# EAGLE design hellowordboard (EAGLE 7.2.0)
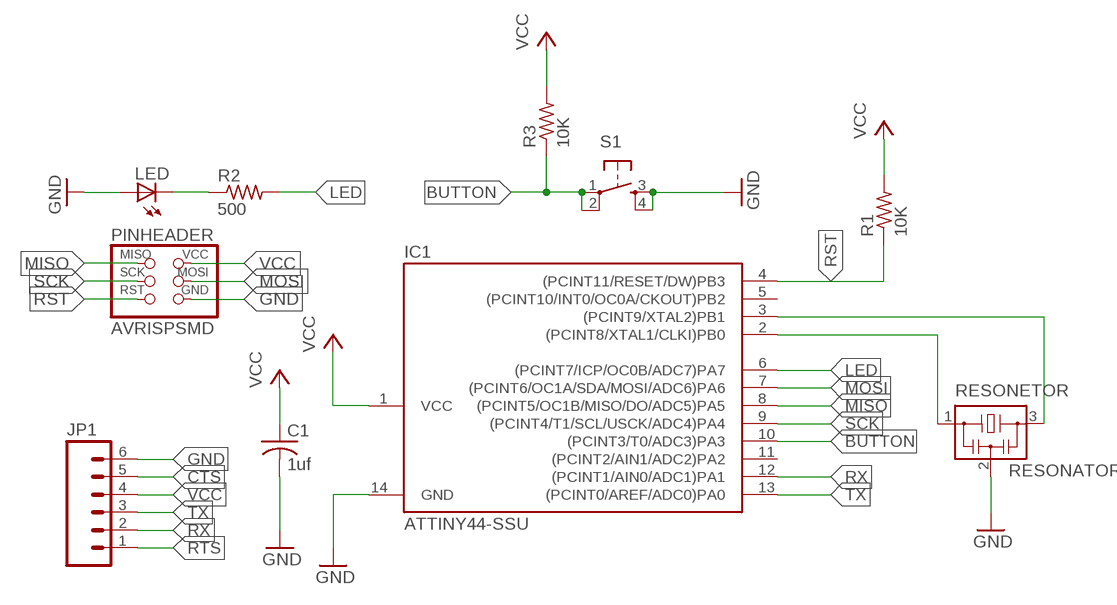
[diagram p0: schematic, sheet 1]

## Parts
C1  1uf  C-USC1206  [C1206]
IC1  ATTINY44-SSU  [SOIC14]
JP1  M06SMD  [1X06-SMD]
LED  LED1206  [1206]
PINHEADER  AVRISPSMD  [2X03SMD]
R1  10K  RESISTOR1206  [1206]
R2  500  RESISTOR1206  [1206]
R3  10K  RESISTOR1206  [1206]
RESONETOR  RESONATOR  [EFOBM]
S1  6MM_SWITCH6MM_SWITCH  [6MM_SWITCH]

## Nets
BUTTON: IC1.10((PCINT3/T0/ADC3)PA3) R3.1 S1.1(P) S1.2(P1)
CTS: JP1.5
GND: C1.2 IC1.14(GND) JP1.6 LED.1(A) PINHEADER.6(GND) RESONETOR.2 S1.3(S) S1.4(S1)
LED: IC1.6((PCINT7/ICP/OC0B/ADC7)PA7) R2.2
MISO: IC1.8((PCINT5/OC1B/MISO/DO/ADC5)PA5) PINHEADER.1(MISO)
MOSI: IC1.7((PCINT6/OC1A/SDA/MOSI/ADC6)PA6) PINHEADER.4(MOSI)
N$2: LED.2(C) R2.1
N$9: IC1.2((PCINT8/XTAL1/CLKI)PB0) RESONETOR.1
N$10: IC1.3((PCINT9/XTAL2)PB1) RESONETOR.3
RST: IC1.4((PCINT11/RESET/DW)PB3) PINHEADER.5(RST) R1.1
RTS: JP1.1
RX: IC1.12((PCINT1/AIN0/ADC1)PA1) JP1.2
SCK: IC1.9((PCINT4/T1/SCL/USCK/ADC4)PA4) PINHEADER.3(SCK)
TX: IC1.13((PCINT0/AREF/ADC0)PA0) JP1.3
VCC: C1.1 IC1.1(VCC) JP1.4 PINHEADER.2(VCC) R1.2 R3.2
Unconnected: IC1.5((PCINT10/INT0/OC0A/CKOUT)PB2) IC1.11((PCINT2/AIN1/ADC2)PA2)

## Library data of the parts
C1 = 01_adafruit:C-US: CAPACITOR, American symbol
IC1 = 01_FAB_Hello:ATTINY44
JP1 = 01_SparkFun:M06: Header 6 Standard 6-pin 0.1" header. Use with straight break away headers (SKU : PRT-00116), right angle break away headers (PRT-00553), swiss pins (PRT-00743), machine pins (PRT-00117), and female headers (PRT-00115). Molex polarized connector foot print use with SKU : PRT-08094 with associated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
LED = 01_FAB_Hello:LED
PINHEADER = 01_FAB_Hello:AVRISP
R1-R3 = 01_FAB_Hello:RESISTOR
RESONETOR = 01_fab:RESONATOR
S1 = 01_FAB_Hello:6MM_SWITCH: OMRON SWITCH

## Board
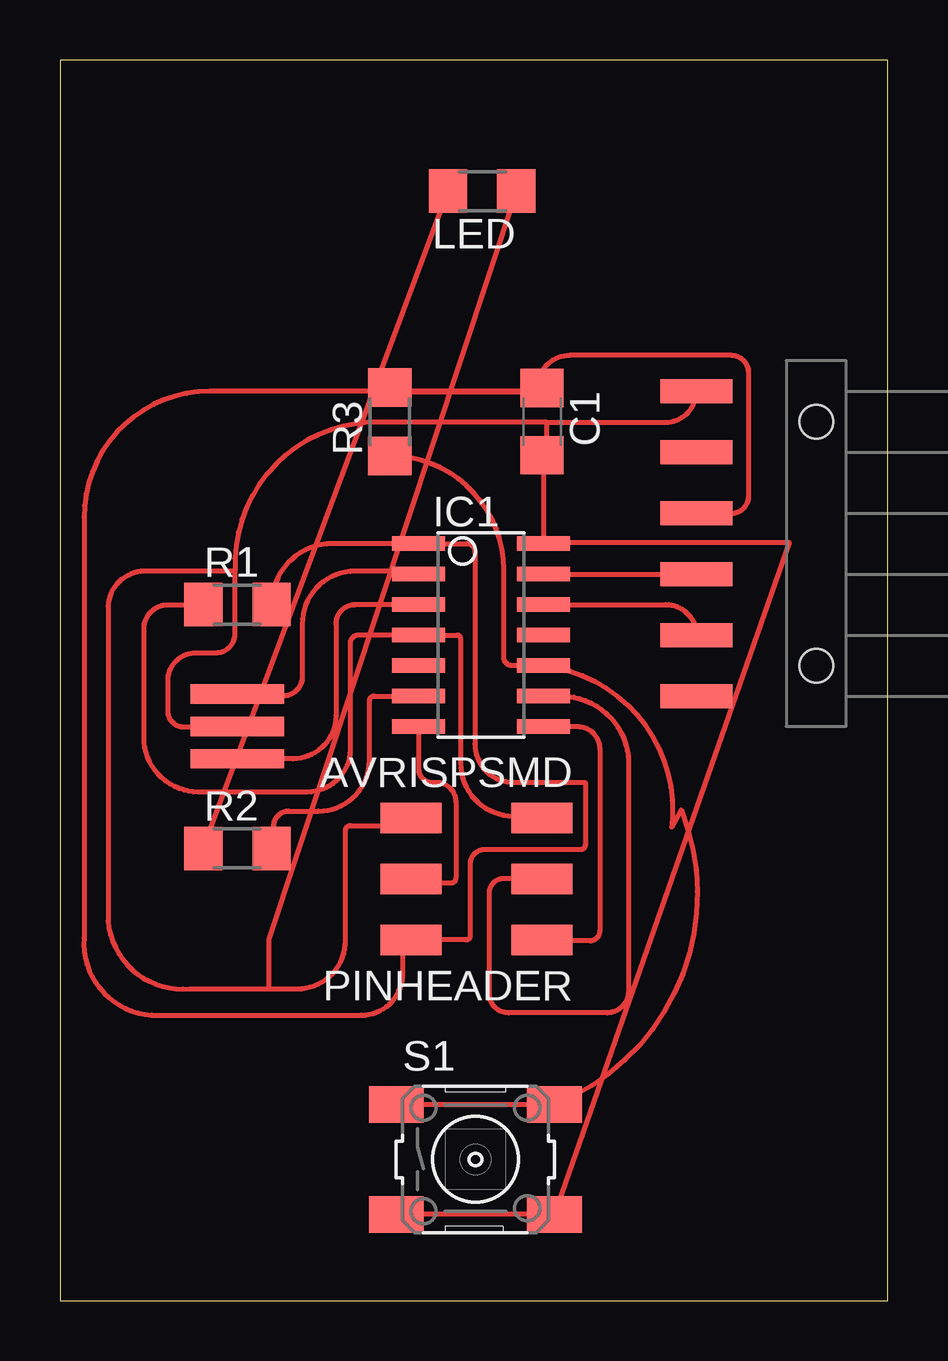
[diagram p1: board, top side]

Size 34.5 x 51.7 mm. Coordinates in mm from the lower left corner, seen from the top.
Outline: 0,0 34.5,0 34.5,51.7 0,51.7 0,0
Copper layers (1*16): Top 0.035mm / dielectric 1.5mm / Bottom 0.035mm
Design rules "default": minimum track width 10mil, minimum drill 24mil, track to track 8mil, track to pad 8mil, pad to pad 8mil, via to via 8mil, smd to smd 8mil, copper to edge 40mil, drill to drill 8mil, minimum pad ring 10mil, minimum via ring 8mil, stop-mask expansion 4mil, vias tented up to drill 0mil, thermal gap 10mil

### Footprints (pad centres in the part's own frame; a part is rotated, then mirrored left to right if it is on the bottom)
C1206 = smd 1.6 x 1.8: 1 -1.4,0; 2 1.4,0
SOIC14 = smd 0.61 x 2.21: 1 -3.81,-2.603; 2 -2.54,-2.603; 3 -1.27,-2.603; 4 0,-2.603; 5 1.27,-2.603; 6 2.54,-2.603; 7 3.81,-2.603; 8 3.81,2.603; 9 2.54,2.603; 10 1.27,2.603; 11 0,2.603; 12 -1.27,2.603; 13 -2.54,2.603; 14 -3.81,2.603
1X06-SMD = smd 1 x 3: 1 -6.35,5; 2 -3.81,5; 3 -1.27,5; 4 1.27,5; 5 3.81,5; 6 6.35,5 | hole 1.4: -5.08,0; 5.08,0
1206 = smd 1.6 x 1.803: 1 -1.422,0; 2 1.422,0
2X03SMD = smd 2.54 x 1.27: 1 -2.54,2.54; 2 2.92,2.54; 3 -2.54,0; 4 2.92,0; 5 -2.54,-2.54; 6 2.92,-2.54
EFOBM = smd 0.8 x 3.9: 1 -1.35,0; 2 0,0; 3 1.35,0
6MM_SWITCH = smd 2.286 x 1.524: 1 -3.302,2.286; 2 3.302,2.286; 3 -3.302,-2.286; 4 3.302,-2.286

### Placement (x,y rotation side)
C1  20.1,36.63 270 top
IC1  17.56,27.74 270 top
JP1  31.53,31.55 90 top
LED  17.6,46.24 180 top
PINHEADER  17.56,17.58 180 top
R1  7.4,29.01 0 top
R2  7.4,18.85 0 top
R3  13.75,36.63 90 top
RESONETOR  7.4,23.93 270 top
S1  17.32,5.89 0 top

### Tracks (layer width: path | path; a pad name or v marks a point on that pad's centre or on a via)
BUTTON
  Top 0.2: S1.1 S1.2 arc90 25.9,20.46 25.5,19.73 arc90 IC1.10 18.83,26.47 arc-90 18.5,26.8 18.5,30.46 arc90 R3.1
  Top 0.254: 13.8,34.9 R3.1
GND
  Top 0.2: 7.3,30.4 arc-90 12.9,36.6 20.3,36.6 | 7.3,30.4 3.65,30.4 arc90 2,28.95 2,15.82 arc90 5.42,13 8.7,13 | S1.3 S1.4 30.41,31.6 20.21,31.6 IC1.14 20.16,35.17 C1.2 | 20.3,35.4 20.3,36.6 | 7.3,23.9 5.17,23.9 arc-90 4.5,24.57 4.5,25.83 arc-90 5.67,27 6.5,27 arc90 7.3,27.8 7.3,30.4 | 20.3,36.6 25.23,36.6 arc90 JP1.6 | 8.7,13 9.9,13 arc90 11.9,15 11.9,19.6 arc-90 12.1,19.8 14.32,19.8 arc90 PINHEADER.6 | LED.1 8.7,15.04 8.7,13
  Top 0.254: 13.8,19.9 14.3,19.9 PINHEADER.6 | 20.3,34.9 C1.2 20.3,35.4 | 7.3,23.9 RESONETOR.2
  Top 0.3: 13.64,19.9 14.64,19.9 PINHEADER.6
LED
  Top 0.2: R2.2 8.9,18.85 8.9,19.77 arc-90 9.53,20.4 10.77,20.4 arc90 12.9,22.53 12.9,25 arc-90 13.1,25.2 IC1.6
MISO
  Top 0.2: IC1.8 21.57,23.93 arc-90 22.5,23 22.5,15.4 arc-90 22.1,15 20.14,15 arc-90 PINHEADER.1
MOSI
  Top 0.2: IC1.7 14.96,22.14 arc90 15.5,21.6 15.7,21.6 arc-90 16.5,20.8 16.5,17.6 arc-90 16.3,17.4 14.82,17.4 arc-90 PINHEADER.4
N$2
  Top 0.2: R2.1 LED.2
N$9
  Top 0.2: 14.8,30.4 12.3,30.4 arc90 10.1,28.2 10.1,26 arc-90 9.3,25.2 7.48,25.2 arc-90 RESONETOR.1
  Top 0.254: 14.8,30.4 IC1.2
N$10
  Top 0.2: IC1.3 arc-90 14.95,29 12.3,29 arc90 11.5,28.2 11.5,24.38 arc-90 9.7,22.58 RESONETOR.3
RST
  Top 0.2: PINHEADER.5 arc90 20.02,20.2 18.9,20.2 arc-90 16.7,22.4 16.7,27.6 arc90 16.56,27.74 IC1.4 12.44,27.74 arc90 12.1,27.4 12.1,22.99 arc-90 10.31,21.2 5.78,21.2 arc-90 3.5,23.48 3.5,28 arc-90 4.5,29 5.97,29 arc90 R1.1
RX
  Top 0.2: IC1.12 25.26,29.01 arc-90 JP1.2
SCK
  Top 0.2: IC1.9 20.9,25.2 arc-90 23.7,22.4 23.7,12.89 arc-90 22.81,12 18.7,12 arc-90 17.9,12.8 17.9,17 arc-90 18.5,17.6 20.08,17.6 arc-90 PINHEADER.3
TX
  Top 0.2: 20.3,30.2 20.38,30.28 JP1.3
  Top 0.254: 20.3,30.2 IC1.13 | 26.3,30.4 JP1.3
  Top 0.406: 26.73,30.2 JP1.3
VCC
  Top 0.2: 14.3,37.9 6.25,37.9 arc90 1,32.65 1,15.12 arc90 3.82,11.9 12.55,11.9 arc90 14.3,13.65 14.3,14.6 14.64,14.6 PINHEADER.2 16.94,15.04 arc90 17.1,15.2 17.1,18.2 arc-90 17.7,18.8 21.7,18.8 arc90 21.9,19 21.9,21.6 18.9,21.6 arc-90 17.3,23.2 17.3,31.2 arc90 16.95,31.55 IC1.1 11.36,31.55 arc90 R1.2 | 20.3,38.03 19.9,38.03 arc-90 21.27,39.4 27.98,39.4 arc-90 28.7,38.68 28.7,33.52 arc-90 27.98,32.8 26.53,32.8 JP1.4
  Top 0.254: C1.1 19.8,37.9 14.3,37.9 13.8,37.9 R3.2 | 26.8,32.9 JP1.4
  Top 0.406: C1.1 20.3,38.03 | 26.53,32.9 JP1.4

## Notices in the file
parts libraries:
01_SparkFun: Licensing: CC v3.0 Share-Alike You are welcome to use this library for commercial purposes.
